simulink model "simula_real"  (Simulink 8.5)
settings: Solver=ode45  StartTime=0.0  StopTime=tf  FixedStep=dt  RelTol=1e-6
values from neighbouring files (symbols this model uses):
  Areal = [zeros(n2,n2) eye(n2); -Pinv*R -Pinv*Q]    [mod_estados_real.m]
  Breal = [zeros(n2,1); Pinv*U]    [mod_estados_real.m]
  Creal = zeros(1,2*n2)    [mod_estados_real.m]
  denK = [1/6 1]    [princi_JL_incerto_prefilt_2a_ordem.m]
  Dreal = 0    [mod_estados_real.m]
  numK = 2.5    [princi_JL_incerto_prefilt_2a_ordem.m]
undefined symbols (not defined in the file or in its folder): tau_pre_filt, w0

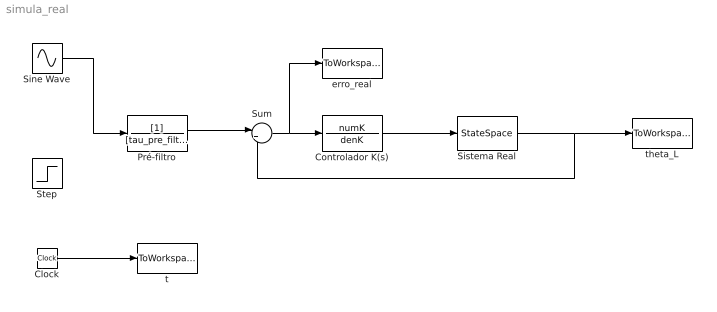
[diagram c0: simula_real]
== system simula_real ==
  Clock : Clock
  Controlador K(s) : TransferFcn  Numerator=numK  Denominator=denK
  Pré-filtro : TransferFcn  Denominator=[tau_pre_filt 1]
  Sine Wave : Sin  Frequency=w0  SampleTime=0
  Sistema Real : StateSpace  A=Areal  B=Breal  C=Creal  D=Dreal  X0=0
  Step : Step  Time=0  SampleTime=0
  Sum : Sum  Inputs=|+-
  erro_real : ToWorkspace  VariableName=erro_real  SampleTime=-1
  t : ToWorkspace  VariableName=t  SampleTime=-1
  theta_L : ToWorkspace  VariableName=theta_L_real  SampleTime=-1
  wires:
  Sum/1 -> erro_real/1, Controlador K(s)/1
  Pré-filtro/1 -> Sum/1
  Clock/1 -> t/1
  Controlador K(s)/1 -> Sistema Real/1
  Sistema Real/1 -> Sum/2, theta_L/1
  Sine Wave/1 -> Pré-filtro/1
